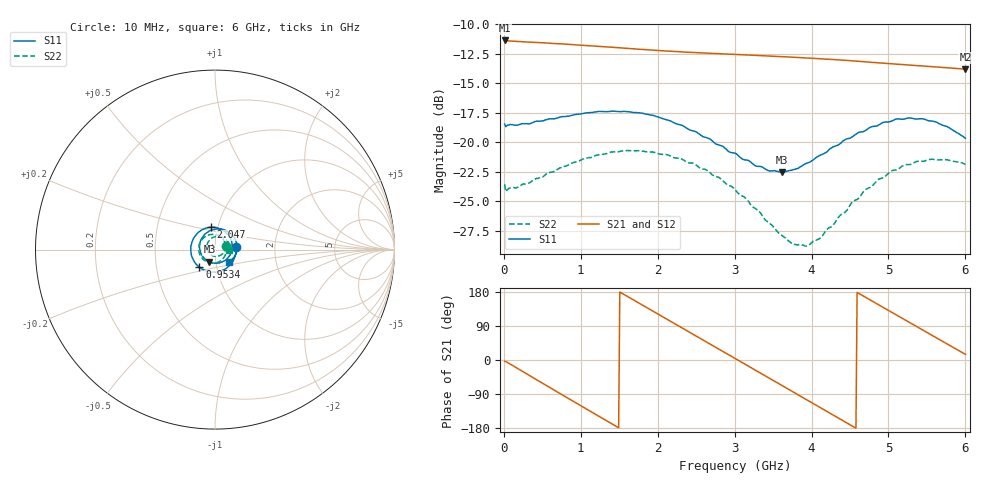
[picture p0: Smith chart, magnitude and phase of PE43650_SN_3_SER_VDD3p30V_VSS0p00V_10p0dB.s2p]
!Keysight Technologies,N5245B,MY57181451,A.13.50.07
!Date: Tuesday, May 07, 2019 08:00:05
!Correction: S11(Full 2 Port(1,2))
!S21(Full 2 Port(1,2))
!S12(Full 2 Port(1,2))
!S22(Full 2 Port(1,2))
!S2P File: Measurements: S11, S21, S12, S22:
# Hz S  dB  R 50
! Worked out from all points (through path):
!   401 points, 10 MHz to 6 GHz, reference 50 ohm
!   highest |S21| = -11.38 dB at 10 MHz (marker M1); lowest = -13.8 dB at 6 GHz (marker M2)
!   group delay of S21, straight-line fit = 326 ps
!   lowest |S11| = -22.6 dB at 3.619 GHz (marker M3), VSWR 1.16, Z = 46.6 - j6.35 ohm
!   |S11| at or under -10 dB: start of sweep to end of sweep
!   |S22| runs from -28.8 to -20.7 dB; largest |S21 - S12| = 0.002
!   S11 on the Smith chart (normalised r, x): 10 MHz: 1.27, +0.03; 953.4 MHz: 0.83, -0.17; 2.047 GHz: 0.93, +0.23; 6 GHz: 1.16, -0.16
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1e7  -18.46 6.3  -11.38 -3.2  -11.43 -3.2  -23.56 17.0
2.496e8  -18.42 -36.8  -11.49 -30.8  -11.54 -30.8  -23.54 -36.2
5.34125e8  -18.13 -76.8  -11.59 -65.0  -11.64 -65.0  -22.78 -76.7
9.53425e8  -17.64 -131.5  -11.76 -115.1  -11.81 -115.1  -21.63 -128.2
1.013325e9  -17.59 -139.1  -11.79 -122.2  -11.84 -122.3  -21.48 -135.4
1.2679e9  -17.39 -169.8  -11.90 -152.4  -11.95 -152.4  -21.03 -163.1
1.5075e9  -17.41 161.7  -12.00 179.3  -12.06 179.3  -20.78 171.5
1.7471e9  -17.51 134.3  -12.12 151.1  -12.18 151.1  -20.72 147.4
2.01665e9  -17.88 103.7  -12.23 119.6  -12.28 119.6  -20.98 120.8
2.0466e9  -17.96 100.1  -12.25 116.0  -12.30 116.1  -21.01 117.6
2.480875e9  -19.08 49.1  -12.40 65.4  -12.46 65.4  -21.85 74.8
2.750425e9  -20.13 16.0  -12.49 33.9  -12.54 34.0  -22.89 46.5
3.005e9  -20.93 -18.6  -12.56 4.2  -12.61 4.3  -23.99 18.8
3.289525e9  -22.03 -61.1  -12.64 -29.1  -12.70 -29.1  -25.69 -17.6
3.618975e9  -22.55 -114.6  -12.75 -67.7  -12.80 -67.6  -27.91 -67.7
3.7837e9  -22.30 -141.8  -12.81 -87.0  -12.85 -87.0  -28.65 -97.4
4.008325e9  -21.57 -176.8  -12.89 -113.3  -12.94 -113.3  -28.47 -140.5
4.277875e9  -20.40 145.6  -12.99 -144.9  -13.05 -144.8  -27.04 173.6
4.517475e9  -19.60 114.4  -13.10 -172.9  -13.15 -172.8  -25.17 139.1
5.01165e9  -18.27 58.2  -13.34 129.5  -13.39 129.7  -22.55 83.6
5.4609e9  -18.04 11.9  -13.55 77.4  -13.60 77.5  -21.60 41.6
6e9  -19.66 -40.1  -13.81 15.0  -13.85 15.1  -21.88 -2.3
